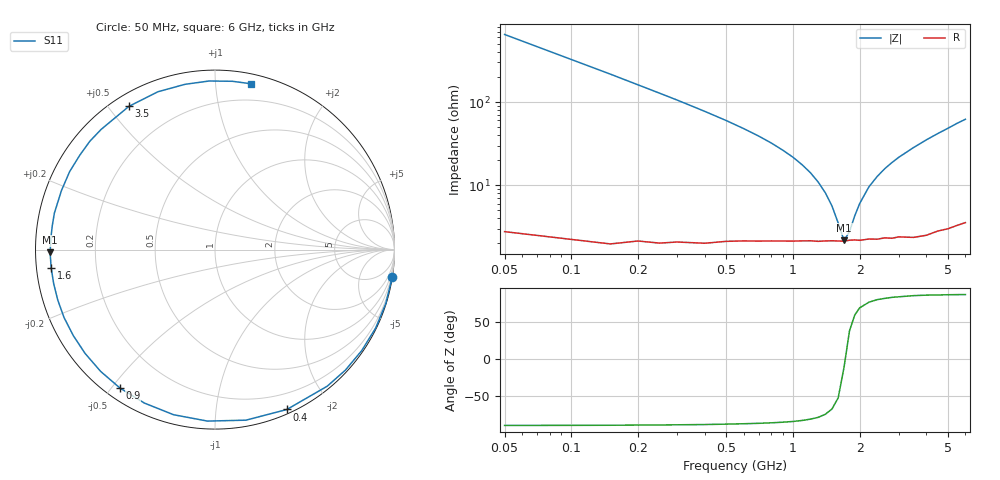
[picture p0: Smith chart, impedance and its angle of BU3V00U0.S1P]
! Infineon Technologies  Discrete & RF Semiconductors
! BB 833
! Si Tuning Diode in SOD323
! VR = 3 V
! S-Parameters:  June  1999
# GHz  S  MA  R  50
!  f  S11
! GHz  MAG  ANG
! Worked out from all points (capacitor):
!   34 points, 50 MHz to 6 GHz, reference 50 ohm
!   read as one part to ground: C = 4.88 pF near 50 MHz
!   lowest |Z| = 2.16 ohm at 1.7 GHz (marker M1)
!   series resonance near 1.72 GHz, so ESL is about 1.8 nH
!   S11 on the Smith chart (normalised r, x): 50 MHz: 0, -13; 400 MHz: 0.04, -1.55; 900 MHz: 0.04, -0.53; 1.6 GHz: 0.04, -0.06; 3.5 GHz: 0.05, +0.56; 6 GHz: 0.07, +1.24
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0.05  0.9993 -8.8
0.1  0.9979 -17.5
0.15  0.996 -26.0
0.25  0.9894 -42.7
0.3  0.985 -50.6
0.4  0.9766 -65.8
0.5  0.9659 -79.7
0.6  0.9564 -92.5
0.7  0.9485 -104.1
0.8  0.9412 -114.7
0.9  0.9354 -124.5
1  0.9309 -133.2
1.1  0.9266 -141.4
1.2  0.9235 -148.8
1.4  0.92 -162.2
1.6  0.9185 -173.6
1.7  0.9188 -179.0
2  0.9177 167.2
2.2  0.9166 159.0
2.4  0.9191 151.8
2.6  0.9188 145.1
3  0.9225 133.4
3.5  0.9311 121.0
4  0.9352 109.9
4.5  0.9359 100.3
5  0.9399 92.0
5.5  0.9428 84.1
6  0.9456 77.7
